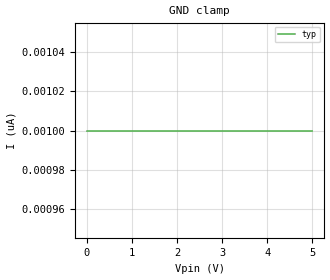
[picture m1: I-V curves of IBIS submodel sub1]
| Ibis file to test add submodel implementation (Bird 48.4)
| Also tests fix for bug 25 (Keyword in Notes etc)
| Also tests Bird 46.1 (filename restrictions relaxed)
| Also tests Bird 51 (3-state_ECL model type)
[IBIS Ver] 3.2
[File Name] addsubmodel.ibs
[File Rev]  hand crafted
| fix for bug 25
[Notes] this is the note the following keywords should not cause a problem
   [Source]
   [Component]
[Source] this is the source.
   [Notes]
[Component] try
[Manufacturer] none
[Package]
R_pkg	1	NA	NA
L_pkg   1n	NA	NA
C_pkg	1f	NA	NA
[Pin] signal_name model_name
1 vcc POWER
   [Model]
| **********  check the Input Model Type ******************
[Model] tryInput
Model_type Input
Vinl = .2
Vinh =  4
C_comp 1f NA NA
| ... junk after the keyword
[Add Submodel]  extradata
[Add Submodel]
| ... no mode specified
sub0
|... cannot be Driving for Input
sub1	Driving
| ... should be OK
sub2   Non-Driving
| ... check case
sub3   non-driving
| ... should be OK
sub4   All
| ... invalid mode
sub5   junk
| ... extra data after mode
sub6   All   extradata
| ... long sub model name
Averyveryveryveryveryveryverylongsubmodelname All
| ... repeated submodel name (should be OK)
sub6   All
[Voltage Range] 5   NA   NA
| **********  check the Terminator Model Type ******************
[Model] tryTerminator
Model_type Terminator
C_comp 1f NA NA
[Add Submodel]
| ... this will be an error
sub1   Driving
| ... this should be OK
sub2   Non-Driving
sub3   All
[Voltage Range] 5   NA   NA
| **********  check the Input_ECL Model Type ******************
[Model] tryInput_ECL
Model_type Input_ECL
Vinl = .2
Vinh = .4
C_comp 1f NA NA
[Add Submodel]
| ... this will be an error
sub1   Driving
| ... this should be OK
sub2   Non-Driving
sub3   All
[Voltage Range] 5   NA   NA
| **********  check the Output Model Type *************
[Model] tryOutput
Model_type Output
C_comp 1f NA NA
[Add Submodel]
sub1   Driving
| ... this will be an error
sub2   Non-Driving
sub3   All
[Voltage Range] 5   NA   NA
[Ramp]
dV/dt_r		1/1n   NA   NA
dV/dt_f		1/1n   NA   NA
| **********  check the Output_ECL Model Type *************
[Model] tryOutput_ECL
Model_type Output_ECL
C_comp 1f NA NA
[Add Submodel]
sub1   Driving
| ... this will be an error
sub2   Non-Driving
sub3   All
[Voltage Range] 5   NA   NA
[Ramp]
dV/dt_r		1/1n   NA   NA
dV/dt_f		1/1n   NA   NA
| **********  check the Open_Drain Model Type *************
[Model] tryOpen_drain
Model_type Open_drain
C_comp 1f NA NA
[Add Submodel]
sub1   Driving
| ... this will be an error
sub2   Non-Driving
sub3   All
[Voltage Range] 5   NA   NA
[Ramp]
dV/dt_r		1/1n   NA   NA
dV/dt_f		1/1n   NA   NA
| **********  check the Open_sink Model Type *************
[Model] tryOpen_sink
Model_type Open_sink
C_comp 1f NA NA
[Add Submodel]
sub1   Driving
| ... this will be an error
sub2   Non-Driving
sub3   All
[Voltage Range] 5   NA   NA
[Ramp]
dV/dt_r		1/1n   NA   NA
dV/dt_f		1/1n   NA   NA
| **********  check the Open_source Model Type *************
[Model] tryOpen_source
Model_type Open_source
C_comp 1f NA NA
[Add Submodel]
sub1   Driving
| ... this will be an error
sub2   Non-Driving
sub3   All
[Voltage Range] 5   NA   NA
[Ramp]
dV/dt_r		1/1n   NA   NA
dV/dt_f		1/1n   NA   NA
| **********  check the I/O Model Type *************
[Model] tryI/O
Model_type I/O
Vinl = .2
Vinh =  4
C_comp 1f NA NA
| ... there should be no error
[Add Submodel]
sub1   Driving
sub2   Non-Driving
sub3   All
[Voltage Range] 5   NA   NA
[Ramp]
dV/dt_r		1/1n   NA   NA
dV/dt_f		1/1n   NA   NA
| **********  check the I/O_open_drain Model Type *************
[Model] tryI/O_open_drain
Model_type I/O_open_drain
Vinl = .2
Vinh =  4
C_comp 1f NA NA
| ... there should be no error
[Add Submodel]
sub1   Driving
sub2   Non-Driving
sub3   All
[Voltage Range] 5   NA   NA
[Ramp]
dV/dt_r		1/1n   NA   NA
dV/dt_f		1/1n   NA   NA
| **********  check the I/O_open_source Model Type *************
[Model] tryI/O_open_source
Model_type I/O_open_source
Vinl = .2
Vinh =  4
C_comp 1f NA NA
| ... there should be no error
[Add Submodel]
sub1   Driving
sub2   Non-Driving
sub3   All
[Voltage Range] 5   NA   NA
[Ramp]
dV/dt_r		1/1n   NA   NA
dV/dt_f		1/1n   NA   NA
| **********  check the I/O_open_sink Model Type *************
[Model] tryI/O_open_sink
Model_type I/O_open_sink
Vinl = .2
Vinh =  4
C_comp 1f NA NA
| ... there should be no error
[Add Submodel]
sub1   Driving
sub2   Non-Driving
sub3   All
[Voltage Range] 5   NA   NA
[Ramp]
dV/dt_r		1/1n   NA   NA
dV/dt_f		1/1n   NA   NA
| **********  check the I/O_ECL Model Type *************
[Model] tryI/O_ECL
Model_type I/O_ECL
Vinl = .2
Vinh =  4
C_comp 1f NA NA
| ... there should be no error
[Add Submodel]
sub1   Driving
sub2   Non-Driving
sub3   All
[Voltage Range] 5   NA   NA
[Ramp]
dV/dt_r		1/1n   NA   NA
dV/dt_f		1/1n   NA   NA
| **********  check the 3-state Model Type *************
[Model] try3-state
Model_type 3-state
C_comp 1f NA NA
| ... there should be no error
[Add Submodel]
sub1   Driving
sub2   Non-Driving
sub3   All
[Voltage Range] 5   NA   NA
[Ramp]
dV/dt_r		1/1n   NA   NA
dV/dt_f		1/1n   NA   NA
| **********  check the 3-state_ECL Model Type *************
[Model] try3-state_ECL
Model_type 3-state_ECL
C_comp 1f NA NA
| ... there should be no error
[Add Submodel]
sub1   Driving
sub2   Non-Driving
sub3   All
[Voltage Range] 5   NA   NA
[Ramp]
dV/dt_r		1/1n   NA   NA
dV/dt_f		1/1n   NA   NA
[Model] AddModelPosition1
Model_type Output
C_comp 1f NA NA
[Voltage Range] 5   NA   NA
| ... [Add Model] should be Before other keywords
[Add Submodel]
sub1	Driving
[Ramp]
dV/dt_r		1/1n   NA   NA
dV/dt_f		1/1n   NA   NA
[Model] AddModelPosition2
Model_type Output
C_comp 1f NA NA
| ... [Add Model] should be after MSPEC
[Add Submodel]
sub1	Driving
[Model Spec]
[Voltage Range] 5   NA   NA
[Ramp]
dV/dt_r		1/1n   NA   NA
dV/dt_f		1/1n   NA   NA
| Models and submodels in the file (19): ? (?), tryInput (Input), tryTerminator (Terminator), tryInput_ECL (Input_ECL), tryOutput (Output), tryOutput_ECL (Output_ECL), tryOpen_drain (Open_drain), tryOpen_sink (Open_sink), tryOpen_source (Open_source), tryI/O (I/O), tryI/O_open_drain (I/O_open_drain), tryI/O_open_source (I/O_open_source), tryI/O_open_sink (I/O_open_sink), tryI/O_ECL (I/O_ECL), try3-state (3-state), try3-state_ECL (3-state_ECL), AddModelPosition1 (Output), AddModelPosition2 (Output), sub1 (Dynamic_clamp)
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| ... a dummy submodel
[Submodel] sub1
Submodel_type Dynamic_clamp
[Ramp]
dV/dt_r		1/1n   NA   NA
dV/dt_f		1/1n   NA   NA
[GND Clamp]
0V        1nA        NA         NA
5V        1nA        NA         NA
